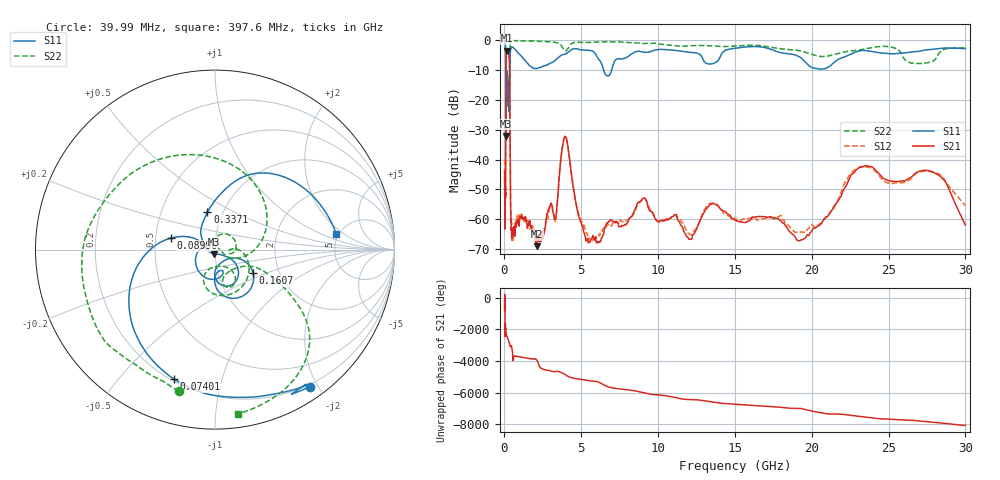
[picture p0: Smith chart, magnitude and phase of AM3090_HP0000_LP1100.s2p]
! Date/Time: Thu, Feb 28, 2019 1:53 PM
! Network Analyzer: Agilent Technologies E8364B Rev: A.07.50.67
! Sweep from 0.010 to 30.000 GHz, 1601 Points, Sweep Type: LOG
! Power Supply: 5.022 V, 0.002 A
# Hz S DB R 50
!freq MagS11 AngS11 MagS21 AngS21 MagS12 AngS12 MagS22 AngS22
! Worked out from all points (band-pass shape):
!   1601 points, 10 MHz to 30 GHz, reference 50 ohm
!   highest |S21| = -3.57 dB at 153.7 MHz (marker M1); lowest = -69.0 dB at 2.094 GHz (marker M2)
!   |S21| within 3 dB of the highest: 99.87 MHz to 319.6 MHz (219.7 MHz wide, 105 % of centre)
!   lowest |S11| = -32.1 dB at 97.94 MHz (marker M3), VSWR 1.05, Z = 49.3 - j2.35 ohm
!   |S11| at or under -10 dB: 88.94 MHz to 349.3 MHz (260.3 MHz wide, 119 % of centre); 6.455 GHz to 6.981 GHz (525.8 MHz wide, 7.83 % of centre)
!   |S22| runs from -34.2 to -0.1 dB; largest |S21 - S12| = 0.012
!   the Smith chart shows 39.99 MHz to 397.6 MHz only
!   S11 on the Smith chart (normalised r, x): 39.99 MHz: 0.17, -1.89; 74.01 MHz: 0.21, -0.71; 89.96 MHz: 0.60, +0.08; 160.7 MHz: 1.47, -0.41; 337.1 MHz: 0.85, +0.37; 397.6 MHz: 4.76, +1.55
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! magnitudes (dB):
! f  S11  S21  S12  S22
! 10 MHz  -0.2  -43.7  -40.1  -0.7
! 38.04 MHz  -0.5  -59.8  -60.0  -1.6
! 39.99 MHz  -0.6  -62.3  -59.2  -1.8
! 74.01 MHz  -2.4  -46.0  -43.1  -4.3
! 89.96 MHz  -11.9  -14.3  -14.2  -12.3
! 97.94 MHz  -32.1  -7.2  -7.2  -33.2
! 113.2 MHz  -13.6  -4.8  -4.8  -19.7
! 144.7 MHz  -19.3  -3.6  -3.6  -21.5
! 153.7 MHz  -14.2  -3.6  -3.6  -17.5
! 160.7 MHz  -12.1  -3.6  -3.6  -15.0
! 337.1 MHz  -13.4  -10.0  -10.0  -8.4
! 397.6 MHz  -3.3  -54.5  -53.8  -0.7
! 550.5 MHz  -2.5  -64.1  -67.2  -0.2
! 2.084 GHz  -9.5  -68.9  -65.7  -0.4
! 2.094 GHz  -9.5  -69.0  -66.8  -0.4
! 3.302 GHz  -6.8  -60.0  -60.7  -0.8
! 3.953 GHz  -4.7  -32.3  -32.2  -3.6
! 5.365 GHz  -3.4  -66.7  -64.6  -0.8
! 7.926 GHz  -5.9  -61.9  -60.5  -0.8
! 19.41 GHz  -6.5  -66.8  -64.3  -3.8
! 23.48 GHz  -3.5  -42.1  -42.5  -2.9
! 30 GHz  -2.8  -61.9  -55.4  -2.6
